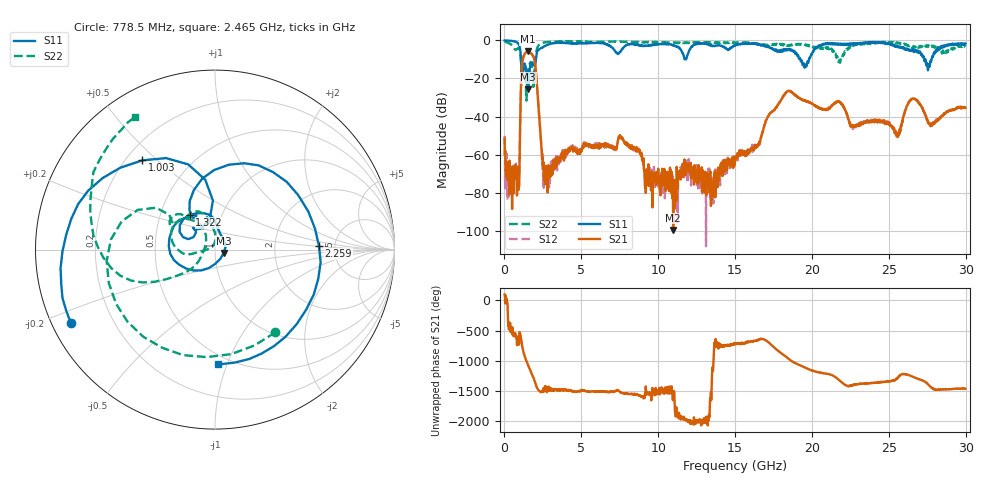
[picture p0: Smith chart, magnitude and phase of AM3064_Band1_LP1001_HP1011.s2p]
# Hz S DB R 50.0
!freq dBS11 angS11 dBS21 angS21 dBS12 angS12 dBS22 angS22
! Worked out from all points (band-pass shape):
!   1600 points, 10 MHz to 29.98 GHz, reference 50 ohm
!   highest |S21| = -5.81 dB at 1.51 GHz (marker M1); lowest = -99.7 dB at 10.98 GHz (marker M2)
!   |S21| within 3 dB of the highest: 1.227 GHz to 1.896 GHz (668.7 MHz wide, 42.8 % of centre)
!   lowest |S11| = -25.7 dB at 1.547 GHz (marker M3), VSWR 1.11, Z = 55 - j2.13 ohm
!   |S11| at or under -10 dB: 1.071 GHz to 2.039 GHz (967.7 MHz wide, 62.2 % of centre); 19.24 GHz to 19.81 GHz (564.3 MHz wide, 2.89 % of centre); 27.38 GHz to 27.78 GHz (405 MHz wide, 1.47 % of centre)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
!   |S22| runs from -31.6 to -0.4 dB; largest |S21 - S12| = 0.0077
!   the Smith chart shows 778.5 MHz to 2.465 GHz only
!   S11 on the Smith chart (normalised r, x): 778.5 MHz: 0.05, -0.24; 1.003 GHz: 0.27, +0.45; 1.322 GHz: 0.70, +0.29; 2.259 GHz: 3.74, +0.23; 2.465 GHz: 0.43, -0.93
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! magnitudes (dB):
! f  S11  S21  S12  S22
! 10 MHz  -0.1  -51.5  -50.2  -0.4
! 778.5 MHz  -0.9  -72.4  -71.3  -4.9
! 1.003 GHz  -3.9  -51.3  -50.9  -5.3
! 1.172 GHz  -15.8  -11.1  -11.0  -11.3
! 1.322 GHz  -12.4  -7.1  -7.0  -13.6
! 1.51 GHz  -23.4  -5.8  -5.8  -17.7
! 1.547 GHz  -25.7  -5.9  -5.8  -15.4
! 1.941 GHz  -13.3  -10.1  -10.1  -16.9
! 2.259 GHz  -4.7  -39.6  -39.5  -2.1
! 2.465 GHz  -3.9  -62.4  -65.8  -1.3
! 5.015 GHz  -1.5  -57.5  -57.5  -0.7
! 7.564 GHz  -5.6  -50.8  -50.8  -0.6
! 10 GHz  -2.0  -67.4  -70.0  -1.0
! 10.98 GHz  -2.7  -99.7  -74.1  -1.1
! 15 GHz  -2.7  -63.7  -62.8  -1.4
! 18.38 GHz  -4.8  -26.9  -26.8  -2.8
! 19.99 GHz  -7.5  -33.2  -33.2  -3.1
! 25 GHz  -1.5  -43.9  -43.6  -1.0
! 25.61 GHz  -3.2  -50.3  -48.3  -1.4
! 26.59 GHz  -5.5  -30.7  -30.5  -3.4
! 27.56 GHz  -15.2  -42.8  -42.7  -2.6
! 29.98 GHz  -1.6  -35.5  -35.1  -3.1
